(* Logix 5000 AddOnInstructionDefinition export B256_EtoL; software revision 30.00 *)

ADD_ON_INSTRUCTION D_SHL   (* revision 1.0, vendor Ken Fischer, NSWCPD, C512 *)
// DINT bit shift left of the 32-bit argument Inp_A by Inp_B bits with paddding by zeros on the right
// Revision note:
// Rev1.0: TBD - Initial Release
VAR_IN_OUT
   Inp_A : DINT; {required}   // 64-bit Integer to be right circular rotated
END_VAR
VAR_INPUT
   Inp_B : INT; {required}   // Number of bits to shift
END_VAR
VAR_IN_OUT
   Out : DINT; {required}   // Result
END_VAR
VAR
   Wrk_InpA : DINT[2];
   Source_Bit : BOOL;
   ONS : BOOL;
   BSL_Cntrl : CONTROL := (LEN := 32);
END_VAR

ROUTINE Logic   (* ladder *)
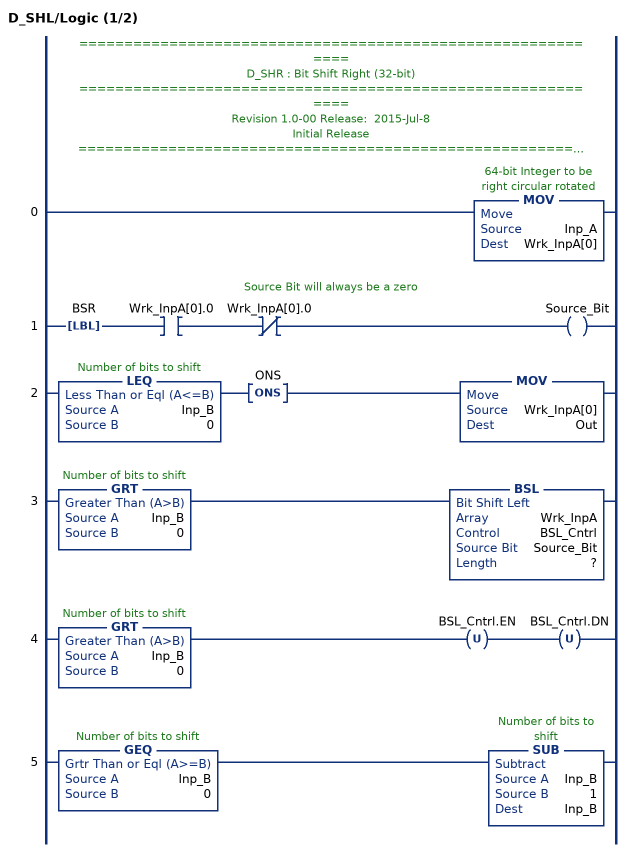
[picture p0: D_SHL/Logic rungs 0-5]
   // ============================================================
   // D_SHR : Bit Shift Right (32-bit)
   // ============================================================
   // Revision 1.0-00 Release:  2015-Jul-8
   // Initial Release
   // ============================================================
   // Performs a left bit shift of the 32-bit argument Inp_A by the
   // number of bits defined in the 16-bit argument Inp_B, with padding by zeros.
   0: MOV(Inp_A,Wrk_InpA[0]);
   // Source Bit will always be a zero
   1: LBL(BSR)XIC(Wrk_InpA[0].0)XIO(Wrk_InpA[0].0)OTE(Source_Bit);
   2: LEQ(Inp_B,0)ONS(ONS)MOV(Wrk_InpA[0],Out);
   3: GRT(Inp_B,0)BSL(Wrk_InpA,BSL_Cntrl,Source_Bit,?);
   4: GRT(Inp_B,0)OTU(BSL_Cntrl.EN)OTU(BSL_Cntrl.DN);
   5: GEQ(Inp_B,0)SUB(Inp_B,1,Inp_B);
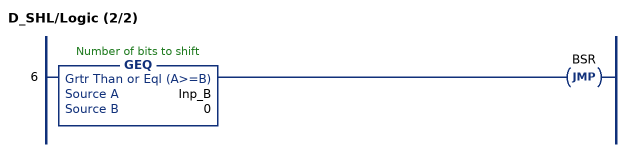
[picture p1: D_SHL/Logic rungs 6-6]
   6: GEQ(Inp_B,0)JMP(BSR);
END_ROUTINE
END_ADD_ON_INSTRUCTION

ADD_ON_INSTRUCTION B256_EtoL   (* revision 1.0 20170916, vendor Kenneth A. Fischer *)
// Convert 256-bit value using 32 8-bit pieces into 256-bit value using 4 64-bit pieces
// Revision note:
// Rev1.0: 20170916 - Initial Release
VAR_IN_OUT
   Inp_E : DINT[32]; {required}
   Out_L : LINT[4]; {required}
END_VAR
VAR
   D_SHL : D_SHL;
   Wrk_Out : DINT[2];
   i : INT;
   j : INT;
   TEMP : DINT;
END_VAR

ROUTINE Logic   (* ladder *)
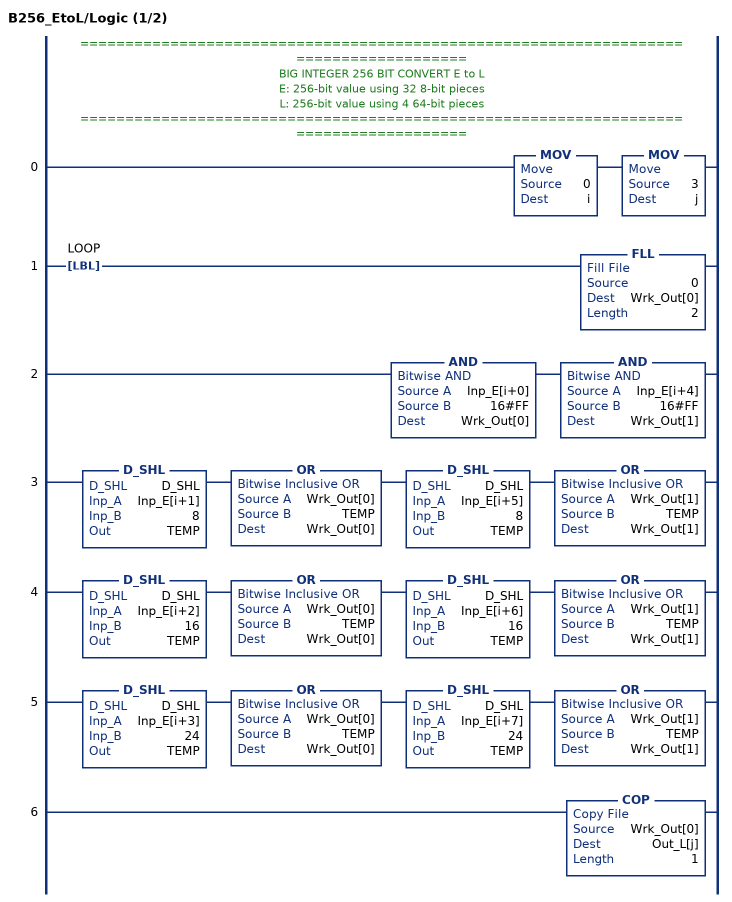
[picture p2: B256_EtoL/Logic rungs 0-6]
   // ======================================================================================
   // BIG INTEGER 256 BIT CONVERT E to L
   // E: 256-bit value using 32 8-bit pieces
   // L: 256-bit value using 4 64-bit pieces
   // ======================================================================================
   0: MOV(0,i)MOV(3,j);
   1: LBL(LOOP)FLL(0,Wrk_Out[0],2);
   2: AND(Inp_E[i+0],16#FF,Wrk_Out[0])AND(Inp_E[i+4],16#FF,Wrk_Out[1]);
   3: D_SHL(D_SHL,Inp_E[i+1],8,TEMP)OR(Wrk_Out[0],TEMP,Wrk_Out[0])D_SHL(D_SHL,Inp_E[i+5],8,TEMP)OR(Wrk_Out[1],TEMP,Wrk_Out[1]);
   4: D_SHL(D_SHL,Inp_E[i+2],16,TEMP)OR(Wrk_Out[0],TEMP,Wrk_Out[0])D_SHL(D_SHL,Inp_E[i+6],16,TEMP)OR(Wrk_Out[1],TEMP,Wrk_Out[1]);
   5: D_SHL(D_SHL,Inp_E[i+3],24,TEMP)OR(Wrk_Out[0],TEMP,Wrk_Out[0])D_SHL(D_SHL,Inp_E[i+7],24,TEMP)OR(Wrk_Out[1],TEMP,Wrk_Out[1]);
   6: COP(Wrk_Out[0],Out_L[j],1);
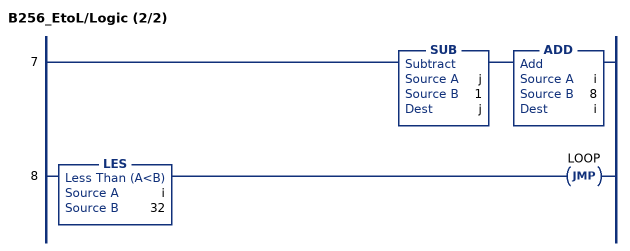
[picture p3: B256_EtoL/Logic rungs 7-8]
   7: SUB(j,1,j)ADD(i,8,i);
   8: LES(i,32)JMP(LOOP);
END_ROUTINE
END_ADD_ON_INSTRUCTION
